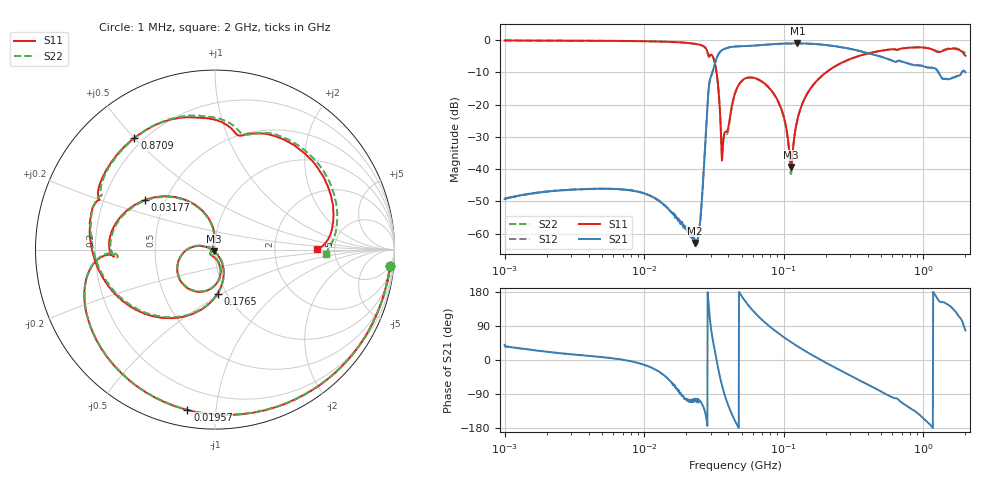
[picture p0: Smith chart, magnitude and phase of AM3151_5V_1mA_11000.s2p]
! Date/Time: Fri Jun 26 11:16:19 2020
! Network Analyzer:  Rev:
! Sweep from 1000000.0 to 2000000000.0, 1601 Points ! Power Supply: 0 V, 0 A
# HZ S DB R 50
!freq MagS11 AngS11 MagS21 AngS21 MagS12 AngS12 MagS22 AngS22
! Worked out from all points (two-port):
!   1601 points, 1 MHz to 2 GHz, reference 50 ohm
!   highest |S21| = -1.05 dB at 125.4 MHz (marker M1); lowest = -62.9 dB at 23 MHz (marker M2)
!   |S21| within 3 dB of the highest: 34.43 MHz to 397 MHz (362.5 MHz wide, 168 % of centre)
!   lowest |S11| = -39.3 dB at 112.9 MHz (marker M3), VSWR 1.02, Z = 49.4 - j0.889 ohm
!   |S11| at or under -10 dB: 32.97 MHz to 201.4 MHz (168.4 MHz wide, 144 % of centre)
!   |S22| runs from -41.5 to -0.2 dB; largest |S21 - S12| = 0.0065
!   S11 on the Smith chart (normalised r, x): 1 MHz: 4, -21; 19.57 MHz: 0.08, -0.84; 31.77 MHz: 0.38, +0.28; 176.5 MHz: 0.91, -0.48; 870.9 MHz: 0.16, +0.50; 2 GHz: 3.66, +0.03
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1000000  -0.16 -5.2  -49.26 40.1  -49.16 35.6  -0.16 -5.2
3555161  -0.24 -17.4  -46.20 13.1  -46.26 12.8  -0.25 -17.5
1.263916e7  -0.47 -62.0  -49.69 -29.7  -49.66 -30.2  -0.48 -62.1
1.956715e7  -0.85 -99.7  -58.05 -100.9  -58.84 -103.5  -0.86 -100.0
2.299717e7  -1.18 -122.0  -62.88 -105.8  -61.53 -106.6  -1.19 -122.4
2.493146e7  -1.48 -137.2  -58.27 -107.1  -58.70 -109.2  -1.50 -137.7
2.88872e7  -4.78 -177.1  -15.58 152.4  -15.55 152.3  -5.12 -177.6
3.176642e7  -6.41 144.6  -7.98 32.1  -7.99 32.1  -6.44 145.2
3.663215e7  -32.71 -152.1  -3.01 -76.1  -3.00 -76.2  -32.49 -160.2
4.493426e7  -16.24 -79.9  -2.02 -162.2  -2.02 -162.2  -16.39 -79.0
5.890834e7  -11.60 -131.2  -1.79 133.8  -1.79 133.8  -11.67 -131.3
8.021973e7  -15.25 -175.4  -1.38 86.7  -1.38 86.7  -15.36 -176.1
9.840022e7  -22.72 164.6  -1.15 61.9  -1.15 61.9  -22.93 162.5
1.129347e8  -39.30 -123.9  -1.08 46.9  -1.07 46.9  -41.42 -115.8
1.253766e8  -24.56 -61.1  -1.05 36.2  -1.06 36.1  -24.54 -58.8
1.589914e8  -14.46 -77.5  -1.21 13.5  -1.19 13.3  -14.45 -77.3
1.765073e8  -12.17 -86.7  -1.33 4.0  -1.34 4.0  -12.21 -86.8
3.151132e8  -5.52 -137.6  -2.95 -45.3  -2.94 -45.4  -5.56 -138.7
5.652395e8  -3.00 169.7  -6.02 -94.2  -5.98 -94.1  -3.00 167.6
8.70922e8  -2.29 125.7  -7.83 -135.0  -7.81 -135.1  -2.30 123.3
1.475665e9  -2.91 62.2  -12.15 147.7  -12.05 147.3  -2.75 59.9
2e9  -4.87 0.3  -10.00 78.2  -10.13 77.6  -4.16 -2.2
